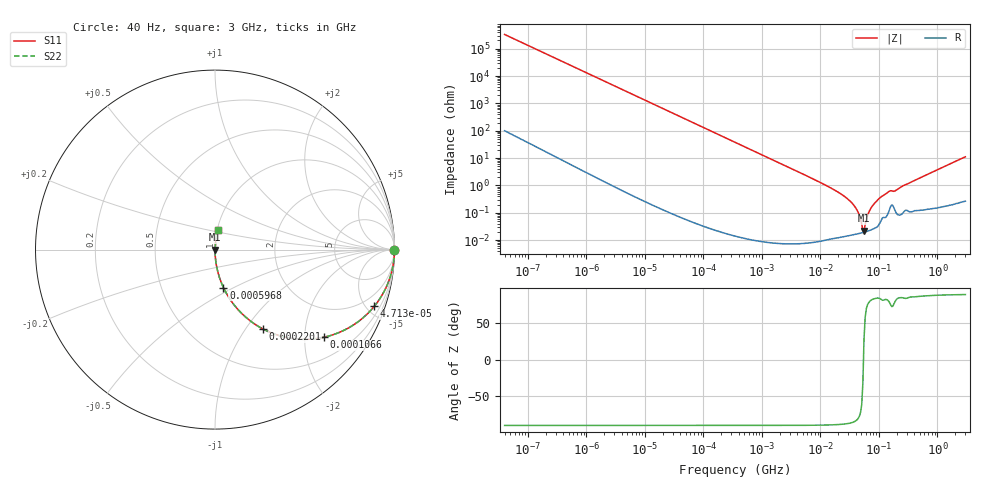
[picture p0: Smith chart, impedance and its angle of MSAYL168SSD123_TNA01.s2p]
! MSAYL168SSD123_TNA01  S-PARAMETER MODEL  ( General Type )
! Model Generated by TAIYO YUDEN Corporation (http://www.ty-top.com)
! Version 2.0
! TAIYO YUDEN Control No. 031107
! Copyright(c) 2003 TAIYO YUDEN CO.,LTD. All Rights Reserved.
! Product Description (link to TY-COMPAS)
! https://ds.yuden.co.jp/TYCOMPAS/or/detail?pn=MSAYL168SSD123KTNA01&u=M
! Products Name : Multilayer Ceramic Capacitors
! Characteristics :
!  Capacitance : 0.012 uF , Rated Voltage : 10V
!  Case Size : 1.6 x 0.8 / 0.063 x 0.031 [mm/inch] , Thickness : 0.8 / 0.031 [mm/inch]
!  (Conditions: Temperature = 25 degC , DC Bias Current/Voltage = 0A / 0V)
! External Node Assignments :
!  1  o---| |---o  2
! GND o---------o GND
! Frequency Range : 40Hz  -  3GHz  [ 401 STEP ]
# MHz S RI R 50
! Freq[MHz].  S11 Real  S11 Imag  S21 Real  S21 Imag  S12 Real  S12 Imag  S22 Real  S22 Imag
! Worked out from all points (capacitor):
!   401 points, 40 Hz to 3 GHz, reference 50 ohm
!   read as one part in series: C = 12 nF near 44 Hz
!   lowest |Z| = 22.2 mohm at 55.54 MHz (marker M1)
!   series resonance near 54.39 MHz, so ESL is about 710 pH
!   S11 on the Smith chart (normalised r, x): 40 Hz: open; 47.13 kHz: 1.00, -5.63; 106.6 kHz: 1.00, -2.49; 220.1 kHz: 1.00, -1.21; 596.8 kHz: 1.00, -0.44; 3 GHz: 1.01, +0.22
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4e-05  1 -0.000301  1.82e-07 0.000301  1.82e-07 0.000301  1 -0.000301
0.000834  1 -0.00629  4.09e-05 0.00629  4.09e-05 0.00629  1 -0.00629
0.017386  0.9831 -0.1288  0.0169 0.1288  0.0169 0.1288  0.9831 -0.1288
0.047134  0.8879 -0.3154  0.1121 0.3154  0.1121 0.3154  0.8879 -0.3154
0.106589  0.6078 -0.4881  0.3922 0.4881  0.3922 0.4881  0.6078 -0.4881
0.220148  0.2665 -0.442  0.7335 0.442  0.7335 0.442  0.2665 -0.442
0.362475  0.1182 -0.3227  0.8818 0.3227  0.8818 0.3227  0.1182 -0.3227
0.596819  0.0472 -0.2118  0.9528 0.2118  0.9528 0.2118  0.0472 -0.2118
7.222098  0.000407 -0.018  0.9996 0.018  0.9996 0.018  0.000407 -0.018
18.71131  0.000159 -0.00623  0.9998 0.00623  0.9998 0.00623  0.000159 -0.00623
30.80834  0.000155 -0.00291  0.9998 0.00291  0.9998 0.00291  0.000155 -0.00291
40.43842  0.000168 -0.00146  0.9998 0.00146  0.9998 0.00146  0.000168 -0.00146
44.27611  0.000174 -0.001  0.9998 0.001  0.9998 0.001  0.000174 -0.001
50.72622  0.000186 -0.000344  0.9998 0.000344  0.9998 0.000344  0.000186 -0.000344
55.54024  0.000195 0.000105  0.9998 -0.000105  0.9998 -0.000105  0.000195 0.000105
58.11596  0.000201 0.000316  0.9998 -0.000316  0.9998 -0.000316  0.000201 0.000316
66.58224  0.000221 0.000987  0.9998 -0.000987  0.9998 -0.000987  0.000221 0.000987
79.8195  0.000261 0.00194  0.9997 -0.00194  0.9997 -0.00194  0.000261 0.00194
104.7695  0.000453 0.00358  0.9995 -0.00358  0.9995 -0.00358  0.000453 0.00358
150.5692  0.00131 0.00603  0.9987 -0.00603  0.9987 -0.00603  0.00131 0.00603
188.875  0.00123 0.00626  0.9988 -0.00626  0.9988 -0.00626  0.00123 0.00626
3000  0.015 0.11  0.985 -0.11  0.985 -0.11  0.015 0.11
